PROGRAM MAIN

VAR CONSTANT	
    cInitSource_DFT			: ST_MA_MultiArray_InitPars := ( eTypeCode := eMA_TypeCode_LREAL, nDims := 1, aDimSizes := [cWindowLength]);
	cInitSource_Spectrum	: ST_MA_MultiArray_InitPars := ( eTypeCode := eMA_TypeCode_LREAL, nDims := 1, aDimSizes := [cBufferLength]);	
END_VAR

VAR
	nInputSelection		: UDINT := 1;						// Switch between hardware and function generator	
	nSample,i,k			: UDINT;
	aEl3632 AT %I*		: ARRAY[1..cOversamples] OF INT;	// Input from hardware e.g. EL3632

	aBufferSignal1		: ARRAY[1..cOversamples] OF LREAL;  // signal part 1 
	aBufferSignal2		: ARRAY[1..cOversamples] OF LREAL;  // signal part 2
	aBuffer				: ARRAY[1..cOversamples] OF LREAL;  // aBufferSignal1 + aBufferSignal2
					
	fbSource_DFT		: FB_CMA_Source :=(	stInitPars := cInitSource_DFT, nOwnID := eID_Source_DFT, 
											aDestIDs := [eID_SparseSpectrum_DFT, eID_RealFFT],
											nResultBuffers := 6);	// Initialize source buffers
	fbSource_Spectrum	: FB_CMA_Source :=(	stInitPars := cInitSource_Spectrum, nOwnID := eID_Source_Spectrum, 
											aDestIDs := [eID_SparseSpectrum_Magnitude, eID_SparseSpectrum_Power, eID_MagnitudeSpectrum, eID_PowerSpectrum],
											nResultBuffers := 8);	// Initialize source buffers
											
	fbSink_DFT			: FB_CMA_Sink := (nOwnID := eID_Sink_DFT);
	fbSink_Magnitude	: FB_CMA_Sink := (nOwnID := eID_Sink_Magnitude);
	fbSink_Power		: FB_CMA_Sink := (nOwnID := eID_Sink_Power);
	
	fbSink_RealFFT				: FB_CMA_Sink := (nOwnID := eID_Sink_RealFFT);
	fbSink_MagnitudeSpectrum	: FB_CMA_Sink := (nOwnID := eID_Sink_MagnitudeSpectrum);
	fbSink_PowerSpectrum		: FB_CMA_Sink := (nOwnID := eID_Sink_PowerSpectrum);
	
	fbFunctionGenerator1	: FB_FunctionGenerator;			// Signal Generator
	fbFunctionGenerator2	: FB_FunctionGenerator;			// Signal Generator
	
	aDFT				: ARRAY[1..cBands] OF ARRAY[1..cBandWidth] OF LCOMPLEX;		// Copy of DFT result
	aMagnitude			: ARRAY[1..cBands] OF ARRAY[1..cBandWidth] OF LREAL;		// Copy of magnitude results
	aPower				: ARRAY[1..cBands] OF ARRAY[1..cBandWidth] OF LREAL;		// Copy of power results
	
	bCalculate			: BOOL;														// Calculation flag for absolute value.
	aDFT_abs			: ARRAY[1..cBands] OF ARRAY[1..cBandWidth] OF LREAL;		// Absolute value of DFT result
	
	aRealFFT			: ARRAY[1..cWindowLength/2+1] OF LCOMPLEX;					// FFT result
	aMagnitudeSpectrum	: ARRAY[1..cWindowLength/2+1] OF LREAL;						// Copy of magnitude spectrum
	aPowerSpectrum		: ARRAY[1..cWindowLength/2+1] OF LREAL;						// Copy of power spectrum
	aRealFFT_abs		: ARRAY[1..cWindowLength/2+1] OF LREAL;						// Absolute value of FFT result
	
	fbErrHist			: FB_HRErrHist; // error monitoring
END_VAR

// Input
CASE nInputSelection OF
	0:  (* input from EL3632 *)
		FOR nSample := 1 TO cOversamples DO
			aBuffer[nSample] := INT_TO_LREAL(aEl3632[nSample]);
		END_FOR
	1:  (* signal generator *)		
		fbFunctionGenerator1(	fFrequency 	:= cSetFrequency[1],
								fAmplitude 	:= cSetAmplitude[1],
								eFunction 	:= E_FunctionType.Sine,
								aSignal		:= aBufferSignal1 );
		fbFunctionGenerator2(	fFrequency 	:= cSetFrequency[2],
								fAmplitude 	:= cSetAmplitude[2],
								eFunction 	:= E_FunctionType.Sine,
								aSignal		:= aBufferSignal2 );
		FOR nSample := 1 TO cOversamples DO
			aBuffer[nSample] := aBufferSignal1[nSample]+aBufferSignal2[nSample];
		END_FOR
END_CASE

// Call source to collect data
CollectData();

// Push results to sink
SinkData();

METHOD CollectData : BOOL
VAR_INPUT
END_VAR
fbSource_DFT.Input1DStd( pDataIn 			:= ADR(aBuffer),
						 nDataInSize 		:= SIZEOF(aBuffer), 
						 eElementType 		:= eMA_TypeCode_LREAL,
						 nOptionPars		:= cCMA_Option_MarkInterruption ); 
IF fbSource_DFT.bError THEN
	fbErrHist.AddError(bErr:=TRUE, hrErrCode:=fbSource_DFT.hrErrorCode, sErrSource:='MAIN.fbSource_DFT'); // error monitoring
	// ToDo: if error
END_IF

fbSource_Spectrum.Input1DStd( pDataIn 			:= ADR(aBuffer),
							 nDataInSize 		:= SIZEOF(aBuffer), 
							 eElementType 		:= eMA_TypeCode_LREAL,
							 nOptionPars		:= cCMA_Option_MarkInterruption ); 
IF fbSource_Spectrum.bError THEN
	fbErrHist.AddError(bErr:=TRUE, hrErrCode:=fbSource_Spectrum.hrErrorCode, sErrSource:='MAIN.fbSource_Spectrum'); // error monitoring
	// ToDo: if error
END_IF
END_METHOD

METHOD SinkData : BOOL
VAR_INPUT
END_VAR
fbSink_DFT.Output1DStd(	pDataOut 		:= ADR(aDFT), 
						nDataOutSize 	:= SIZEOF(aDFT), 
						eElementType 	:= eMA_TypeCode_LCOMPLEX, 
						nOptionPars		:= 0,
						bNewResult		=> bCalculate );
IF fbSink_DFT.bError THEN
	fbErrHist.AddError(bErr:=TRUE, hrErrCode:=fbSink_DFT.hrErrorCode, sErrSource:='MAIN.fbSink_DFT'); // error monitoring
	// ToDo: if error
END_IF

IF bCalculate THEN
	FOR i := 1 TO cBands DO
		FOR k := 1 TO cBandWidth DO
			aDFT_abs[i][k] := SQRT( aDFT[i][k].re * aDFT[i][k].re + aDFT[i][k].im * aDFT[i][k].im );
		END_FOR 
	END_FOR
	bCalculate := FALSE;
END_IF

fbSink_Magnitude.Output1DStd(	pDataOut 		:= ADR(aMagnitude), 
								nDataOutSize 	:= SIZEOF(aMagnitude), 
								eElementType 	:= eMA_TypeCode_LREAL, 
								nOptionPars		:= 0);
IF fbSink_Magnitude.bError THEN
	fbErrHist.AddError(bErr:=TRUE, hrErrCode:=fbSink_Magnitude.hrErrorCode, sErrSource:='MAIN.fbSink_Magnitude'); // error monitoring
	// ToDo: if error
END_IF

fbSink_Power.Output1DStd(	pDataOut 		:= ADR(aPower), 
							nDataOutSize 	:= SIZEOF(aPower), 
							eElementType 	:= eMA_TypeCode_LREAL, 
							nOptionPars		:= 0);
IF fbSink_Power.bError THEN
	fbErrHist.AddError(bErr:=TRUE, hrErrCode:=fbSink_Power.hrErrorCode, sErrSource:='MAIN.fbSink_Power'); // error monitoring
	// ToDo: if error
END_IF

fbSink_RealFFT.Output1DStd(	pDataOut 		:= ADR(aRealFFT), 
							nDataOutSize 	:= SIZEOF(aRealFFT), 
							eElementType 	:= eMA_TypeCode_LCOMPLEX, 
							nOptionPars		:= 0,
							bNewResult		=> bCalculate );
IF fbSink_RealFFT.bError THEN
	fbErrHist.AddError(bErr:=TRUE, hrErrCode:=fbSink_RealFFT.hrErrorCode, sErrSource:='MAIN.fbSink_RealFFT'); // error monitoring
	// ToDo: if error
END_IF

IF bCalculate THEN
	FOR i := 1 TO cWindowLength/2+1 DO
		aRealFFT_abs[i] := SQRT( aRealFFT[i].re * aRealFFT[i].re + aRealFFT[i].im * aRealFFT[i].im );
	END_FOR
	bCalculate := FALSE;
END_IF

fbSink_MagnitudeSpectrum.Output1DStd(	pDataOut 		:= ADR(aMagnitudeSpectrum), 
										nDataOutSize 	:= SIZEOF(aMagnitudeSpectrum), 
										eElementType 	:= eMA_TypeCode_LREAL, 
										nOptionPars		:= 0);
IF fbSink_MagnitudeSpectrum.bError THEN
	fbErrHist.AddError(bErr:=TRUE, hrErrCode:=fbSink_MagnitudeSpectrum.hrErrorCode, sErrSource:='MAIN.fbSink_MagnitudeSpectrum'); // error monitoring
	// ToDo: if error
END_IF

fbSink_PowerSpectrum.Output1DStd(	pDataOut 		:= ADR(aPowerSpectrum), 
									nDataOutSize 	:= SIZEOF(aPowerSpectrum), 
									eElementType 	:= eMA_TypeCode_LREAL, 
									nOptionPars		:= 0);
IF fbSink_PowerSpectrum.bError THEN
	fbErrHist.AddError(bErr:=TRUE, hrErrCode:=fbSink_PowerSpectrum.hrErrorCode, sErrSource:='MAIN.fbSink_PowerSpectrum'); // error monitoring
	// ToDo: if error
END_IF
END_METHOD

END_PROGRAM
